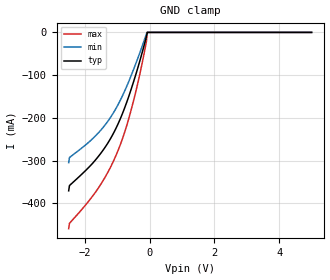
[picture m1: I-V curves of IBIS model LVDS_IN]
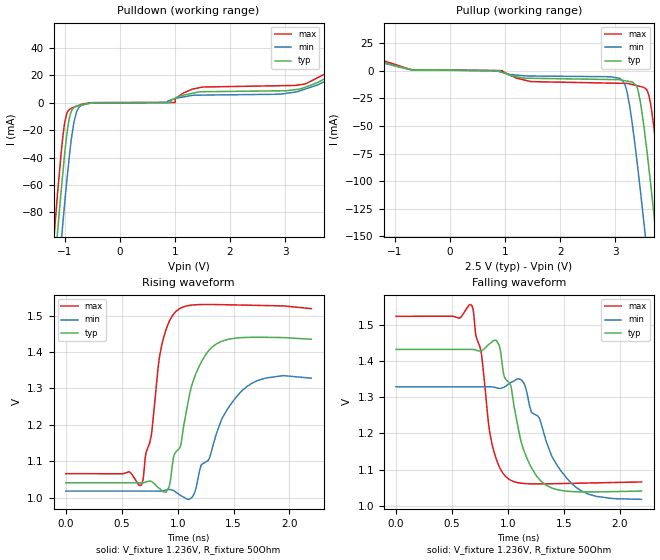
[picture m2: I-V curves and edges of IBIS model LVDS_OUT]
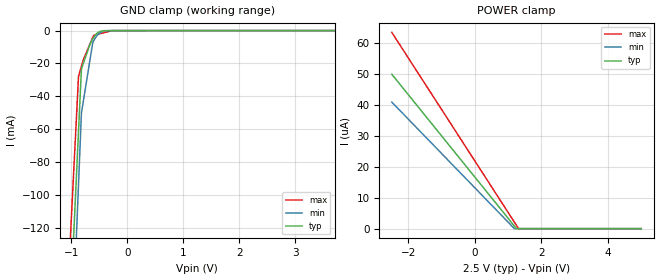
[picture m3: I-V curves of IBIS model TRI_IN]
| Texas Instruments Incorporated
| Dual 1:2 Low Additive Jitter LVDS buffer
| Marketing part#   Voltage Range   Package-type   #pins/pkg drawing
| CDCLVD2102   2.375V-2.625V   QFN   16-pin QFN
[IBIS Ver]   4.0
[File name]   cdclvd2102.ibs
[File Rev]   1.2
[Date]   10/23/2018
[Source]   spectre simulations
   Texas Instruments Incorporated.
   Analog eLab Design Center, HPA
   12500 TI Blvd
   Dallas, TX -75243
   For Support e-mail: elab_scm_ibis@list.ti.com
[Notes]   Revision History:
   Rev 1.2: 10/23/2018
   - TRI_IN model updated to reflect true electrical behavior.
   - VBB_OUT model removed  due  to inaccurary in describing
   termination behavior.
   Rev 1.1: 9/23/2013
   - Updated LVDS_IN to correct POWER and GROUND Clamp models.
   Rev 1.0: 07/06/2010
   - C_comp although listed in numberical order of value are obtained from varying PVT conditions.
   For PVT conditions for eachspecific value, refer to the buffer description under repective [Model].
   IBIS model user is responsible for using appropriate C_comp to simulate for Signal Integrity.
   - TISPice simulation of Clamp current does not match silicon
   - POWER and GND clamp for TRI_IN, D_REB_IN non-monotonic due circuit design
   - GND clamp for LVDS_IN non-monotonic due to circuit design
   - LVDS_OUT pullup/pulldown non-monotonic as a result of circuit design
[Disclaimer] This model is designed as an aid for customers of Texas Instruments.
 TI and its licensors and suppliers make no warranties, either expressed
 or implied, with respect to this  model, including the warranties of
 merchantability or fitness for a particular purpose.
 The model is provided solely on an "as is" basis. The entire risk as to
 its quality and performance is with the customer.
[Copyright] (C)Copyright 2013 Texas Instruments Incorporated.
   All rights reserved.
|   Component CDCLVD2102
[Component]   CDCLVD2102
[Manufacturer]  Texas Instruments Incorporated
[Package]   |QFN (RGT) 16-pin
|   typ   min   max
R_pkg   0.0658   0.0248   0.0806
L_pkg   0.8404nH   0.6985nH   1.0659nH
C_pkg   0.1111pF   0.1026pF   0.1480pF
[Pin]   signal_name   model_name   R_pin   L_pin   C_pin
1   GND   GND   0.0363   0.7137p  0.1279p
2   EN   TRI_IN   0.0650   0.8703p  0.1099p
3   INP1   LVDS_IN   0.0647   0.8300p  0.1088p
4   INN1   LVDS_IN   0.0737   0.9642p  0.1067p
5   VCC   POWER   0.0248   0.6985p  0.1493p
6   INP0   LVDS_IN   0.0658   0.8427p  0.1111p
7   INN0   LVDS_IN   0.0658   0.8402p  0.1099p
8   VAC_REF   NC   0.0770   1.0056p  0.1085p
9   OUTP0   LVDS_OUT   0.0770   1.0051n  0.1085p
10   OUTN0   LVDS_OUT   0.0658   0.8370n  0.1097p
11   OUTP1   LVDS_OUT   0.0658   0.8370n  0.1097p
12   OUTN1   LVDS_OUT   0.0770   1.0051n  0.1085p
13   OUTP2   LVDS_OUT   0.0770   1.0058n  0.1085p
14   OUTN2   LVDS_OUT   0.0658   0.8404n  0.1099p
15   OUTP3   LVDS_OUT   0.0658   0.8429n  0.1100p
16   OUTN3   LVDS_OUT   0.0770   1.0120n  0.1094p
[Diff_pin]   inv_pin   vdiff   tdelay_typ   tdelay_min   tdelay_max
| The 'OUTPx' pin is Diff_pin and the 'OUTNx' pin is the inv_pin
| The 'INPx' pin is Diff_pin and the 'INNx' pin is the inv_pin
3   4   0.200   0 0 0
6   7   0.200   0 0 0
9   10   0.200   0 0 0
11   12   0.200   0 0 0
13   14   0.200   0 0 0
15   16   0.200   0 0 0
| Models and submodels in the file (3): LVDS_IN (Input), LVDS_OUT (Output), TRI_IN (Input)
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|   LVDS Input Model
[Model]   LVDS_IN
Model_type   Input
|Signals   INN0,INP0,INN1,INP1
Vinh = 1.6
Vinl = 0.3
| variable   typ   min   max
|   (nom PVT)   (slow PVT)   (fast PVT)
C_comp   3.121pF   2.849pF   3.193pF
| Ccomp comes from PVT, calculated at 800MHz.
| Nom PVT is nom process, 2.5V, 25C
| slow PVT is weak process, 2.375V, 105C
| Fast process is strong process, 2.625V, -40C
|   typ   min   max
[Voltage Range]   2.5   2.375   2.625
[Temperature Range]   25   105   -40
[Power Clamp Reference]   2.5   2.375   2.625
[GND Clamp Reference]   0   0   0
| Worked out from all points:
|   GND clamp passes 1 mA (typ) near -0.08 V on its own axis
[GND Clamp]
|   Voltage   I(typ)   I(min)   I(max)
-2.5V     -370.8mA   -304.9mA   -459.4mA
-2.475V   -358.5mA   -293mA     -446.8mA
-1.9V     -317.5mA   -258.4mA   -396.7mA
-1.5V     -282.1mA   -228.1mA   -354.5mA
-1.225V   -250.8mA   -200.9mA   -318mA
-975mV    -214.1mA   -169mA     -276.3mA
-700mV    -161.8mA   -124.9mA   -216.1mA
-450mV    -104.2mA   -77.57mA   -145.7mA
-150mV    -24.38mA   -14.67mA   -41.36mA
-100mV    -9.871mA   -3.55mA    -21.64mA
-75.01mV  0A         0A         0A
5V        0A         0A         0A
[POWER Clamp]
|   Voltage   I(typ)   I(min)   I(max)
-2.5V     0A         0A         0A
-2.475V   0A         0A         0A
-2.45V    0A         0A         0A
5V        0A         0A         0A
|   LVDS_OUT Model
[Model]   LVDS_OUT
Model_type   Output
| Signals   OUTP0,OUTN0,OUTP1,OUTN1,OUTP2,OUTN2,OUTP3,OUTN3
Polarity   Non-Inverting
Vmeas = 1.25
Vref = 1.25
Cref = 15pF
Rref = 50
| variable   typ   min   max
|   (nom PVT)   (slow PVT)   (fast PVT)
C_comp   1.275pF   1.175pF   1.317pF
| Ccomp comes from PVT corner simulations
| Nom PVT is nom process, 2.5V, 25C
| slow PVT is weak process, 2.375V, 105C
| Fast process is strong process, 2.625V, -40C
[Voltage Range]   2.5   2.375   2.625
[Temperature Range]   25   105   -40
[Pullup Reference]   2.5   2.375   2.625
[Pulldown Reference]   0   0   0
[Power Clamp Reference]   2.5   2.375   2.625
[GND Clamp Reference]   0   0   0
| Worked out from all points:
|   slope of the pulldown table from 0 to 0.375 V, typ, clamps not added: 11.9 kohm
|   slope of the pullup table from 0 to 0.375 V, typ, clamps not added: 2.06 kohm
|   falling waveform, V_fixture 1.236V, R_fixture 50Ohm: 20-80 % time 216ps typ, 313ps min, 114ps max; typ from 1.43 V to 1.04 V
|   rising waveform, V_fixture 1.236V, R_fixture 50Ohm: 20-80 % time 213ps typ, 297ps min, 111ps max; typ from 1.04 V to 1.44 V
[Pulldown]
|   Voltage   I(typ)   I(min)   I(max)
-2.5V     -819.9mA   -841.2mA   -808.9mA
-1.205V   -132.7mA   -170.8mA   -104.8mA
-1.179V   -119.9mA   -157.8mA   -91.4mA
-1.126V   -94.38mA   -132.6mA   -65.81mA
-1.057V   -62.54mA   -100.1mA   -34.83mA
-992.5mV  -35.05mA   -71.07mA   -13.52mA
-904.2mV  -9.792mA   -35.76mA   -4.869mA
-801.5mV  -2.839mA   -9.874mA   -2.967mA
-497.6mV  -107.4uA   -219.6uA   -77.81uA
1.006V    3.123mA    2.958mA    13.07uA
3.348V    10.9mA     9.549mA    13.39mA
4.992V    48.76mA    47.89mA    54.44mA
[Pullup]
|   Voltage   I(typ)   I(min)   I(max)
-2.5V     34.99mA    35.32mA    37.69mA
-673.6mV  752.9uA    742.8uA    631.1uA
3.09V     -8.286mA   -7.075mA   -11.46mA
3.202V    -9.311mA   -16.77mA   -11.57mA
3.31V     -10.29mA   -48.27mA   -12.56mA
3.416V    -18.21mA   -90.66mA   -13.83mA
3.525V    -51.64mA   -139.2mA   -15.42mA
3.637V    -99.27mA   -190.6mA   -28.34mA
3.71V     -133.1mA   -225.4mA   -54.42mA
3.766V    -159.3mA   -252.7mA   -79.01mA
3.928V    -237.8mA   -331.5mA   -155.2mA
4.992V    -776.9mA   -866.8mA   -698.2mA
[Ramp]
R_load = 50
|   typ   min   max
dV/dt_r   0.238696/2.15967e-10   0.19168/3.14155e-10   0.275901/1.13765e-10
dV/dt_f   0.234348/2.15967e-10   0.186163/3.14155e-10   0.274079/1.13765e-10
[Falling Waveform]
V_fixture = 1.236V
V_fixture_min = 1.173V
V_fixture_max = 1.294V
R_fixture = 50Ohm
C_fixture = 0F
|   Time   V(typ)   V(min)   V(max)
0s        1.431V     1.328V     1.523V
675ps     1.432V     1.328V     1.553V
765ps     1.428V     1.328V     1.417V
855ps     1.451V     1.328V     1.176V
920ps     1.445V     1.324V     1.11V
1.01ns    1.34V      1.337V     1.073V
1.135ns   1.16V      1.342V     1.062V
1.305ns   1.066V     1.219V     1.061V
1.62ns    1.039V     1.049V     1.062V
2.195ns   1.041V     1.018V     1.066V
[Rising Waveform]
V_fixture = 1.236V
V_fixture_min = 1.173V
V_fixture_max = 1.294V
R_fixture = 50Ohm
C_fixture = 0F
|   Time   V(typ)   V(min)   V(max)
0s        1.041V     1.018V     1.066V
675ps     1.04V      1.018V     1.035V
765ps     1.044V     1.018V     1.172V
855ps     1.021V     1.018V     1.415V
920ps     1.027V     1.022V     1.481V
1.01ns    1.133V     1.009V     1.518V
1.135ns   1.317V     1.004V     1.53V
1.305ns   1.413V     1.13V      1.531V
1.62ns    1.44V      1.306V     1.529V
2.195ns   1.435V     1.328V     1.52V
|   TRI_IN Input Model
[Model]   TRI_IN
Model_type   Input
Vinl = 0.475
Vinh = 1.8375
|   typ   min   max
C_comp   1.974pF   1.947pF   1.983pF
[Voltage Range]   2.5   2.375   2.625
[Temperature Range]   25   105   -40
[Power Clamp Reference]   2.5   2.375   2.625
[GND Clamp Reference]   0   0   0
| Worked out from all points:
|   GND clamp passes 1 mA (typ) near -0.51 V on its own axis
[GND Clamp]
|   Voltage   I(typ)   I(min)   I(max)
-2.5V     -1.519A    -1.599A    -1.46A
-1.383V   -435.2mA   -519.8mA   -372mA
-872mV    -61.4mA    -93.54mA   -27.86mA
-820mV    -23.3mA    -50.1mA    -21.6mA
-782.5mV  -19.62mA   -42.18mA   -17.41mA
-670mV    -8.564mA   -18.42mA   -8.334mA
-617.5mV  -5.055mA   -7.338mA   -4.098mA
-602.5mV  -4.217mA   -6.329mA   -2.888mA
-497.5mV  -686.1uA   -1.614mA   -1.968mA
-415mV    -96.99uA   -336uA     -1.246mA
-275.7mV  -21.08uA   -26.56uA   -26.45uA
5V        0A         0A         0A
[POWER Clamp]
|   Voltage   I(typ)   I(min)   I(max)
-2.5V     49.93uA    40.92uA    63.45uA
1.183V    882.3nA    41.92nA    2.147uA
1.242V    83.42nA    0A         1.149uA
1.31V     0A         0A         25.11nA
5V        0A         0A         0A
